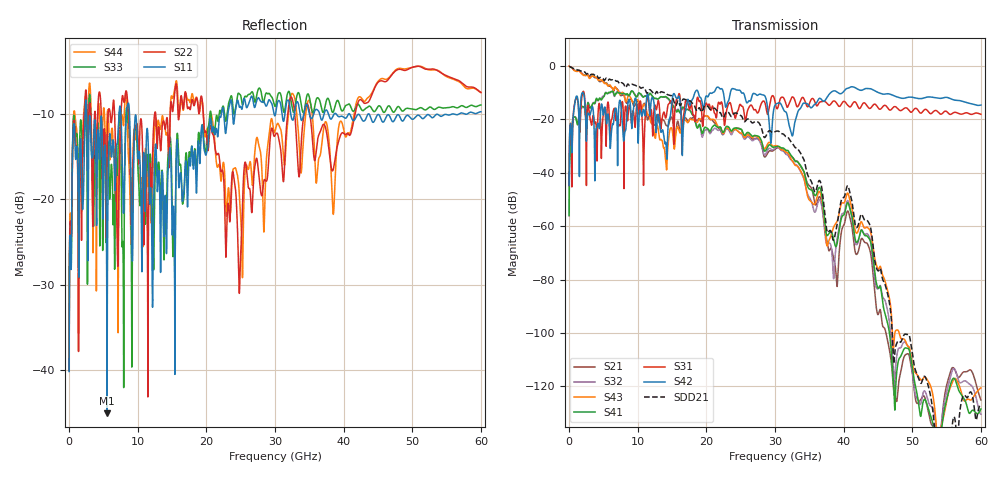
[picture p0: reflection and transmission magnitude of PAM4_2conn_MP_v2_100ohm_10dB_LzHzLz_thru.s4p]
! Info: Touchstone file created by Circ.  Input file=FAB50GbE_2conn_Midplane_Examax_Topo2_v2_100ohm_10dB_LzHzLz.circ
# Hz S RI R 50
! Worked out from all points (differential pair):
!   6000 points, 10 MHz to 60 GHz, reference 50 ohm
!   strongest paths, dB at 10 MHz, 15.01 GHz, 30.01 GHz, 45.01 GHz, 60 GHz:
!     S42: -44.7, -13.0, -14.7, -9.9, -14.7
!     S31: -44.7, -14.2, -13.4, -15.7, -18.1
!     S41: -56.1, -14.3, -30.3, -83.1, -128.5
!     S43: -0.1, -23.9, -29.9, -76.0, -120.6
!     S32: -56.1, -14.3, -30.8, -83.5, -130.4
!     S21: -0.1, -19.4, -31.2, -93.1, -125.1
!   taken as a pair (ports 3,1 in; 4,2 out), SDD21 dB: -0.1, -11.3, -24.6, -76.7, -126.8
!   lowest |S11| = -45.1 dB at 5.54 GHz (marker M1), VSWR 1.01, Z = 49.8 - j0.528 ohm
!   |S11| at or under -10 dB: 2.572 GHz to 7.284 GHz (4.712 GHz wide, 95.6 % of centre); 8.804 GHz to 22.19 GHz (13.39 GHz wide, 86.4 % of centre); 40.84 GHz to 56.85 GHz (16.02 GHz wide, 32.8 % of centre)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
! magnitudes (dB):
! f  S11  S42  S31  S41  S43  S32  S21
! 10 MHz  -40.2  -44.7  -44.7  -56.1  -0.1  -56.1  -0.1
! 5.54 GHz  -45.1  -20.1  -16.3  -10.4  -7.1  -10.3  -6.6
! 32 GHz  -8.5  -21.5  -14.5  -32.1  -33.2  -33.9  -32.8
! 38.94 GHz  -10.0  -9.6  -13.8  -67.5  -58.7  -66.7  -79.3
! 40.62 GHz  -10.1  -8.4  -14.8  -51.3  -47.7  -50.4  -54.3
! 44.8 GHz  -10.3  -9.7  -14.9  -81.5  -74.7  -83.2  -91.2
! 60 GHz  -9.8  -14.7  -18.1  -128.5  -120.6  -130.4  -125.1
